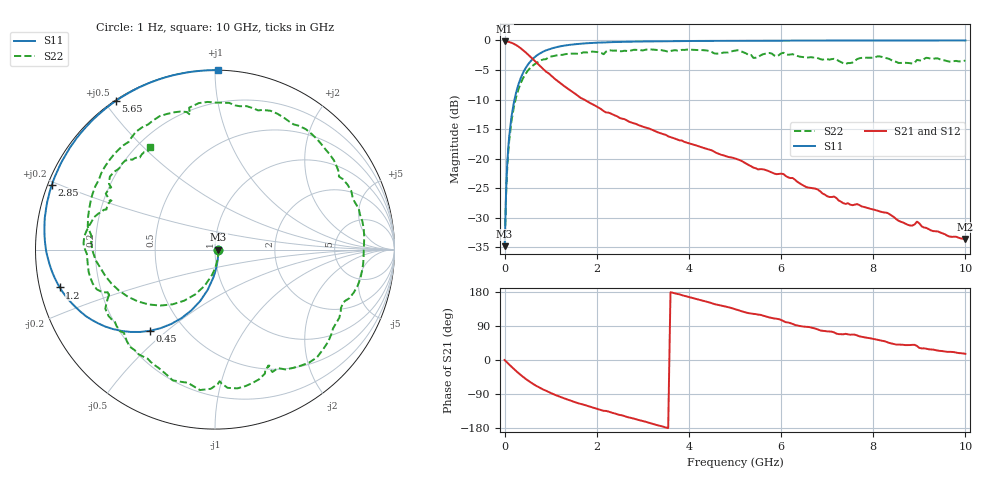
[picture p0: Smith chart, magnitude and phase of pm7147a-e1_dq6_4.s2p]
# GHz S DB R 50
! S-Parameters data
! Freq  dbS11  angS11  dbS21  angS21  dbS12  angS12  dbS22  angS22
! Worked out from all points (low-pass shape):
!   279 points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, 1 Hz to 10 GHz, reference 50 ohm
!   highest |S21| = -0.16 dB at 79.4 Hz (marker M1); lowest = -33.6 dB at 10 GHz (marker M2)
!   |S21| within 3 dB of the highest: start of sweep to 612.8 MHz
!   lowest |S11| = -34.8 dB at 79.4 Hz (marker M3), VSWR 1.04, Z = 51.9 - j3.07e-06 ohm
!   |S11| at or under -10 dB: start of sweep to 215.3 MHz
!   |S22| runs from -34.8 to -1.5 dB; largest |S21 - S12| = 1.1e-11
!   S11 on the Smith chart (normalised r, x): 1 Hz: 1.04, -0.00; 450 MHz: 0.32, -0.44; 1.2 GHz: 0.06, -0.12; 2.85 GHz: 0.01, +0.19; 5.65 GHz: 0.00, +0.54; 10 GHz: 0.00, +1.02
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1e-09  -34.81 -0.0  -0.16 -0.0  -0.16 -0.0  -34.81 -0.0
7.94e-08  -34.81 -0.0  -0.16 -0.0  -0.16 -0.0  -34.81 -0.0
0.03162278  -25.64 -72.5  -0.17 -3.8  -0.17 -3.8  -26.27 -72.2
0.06309573  -20.08 -85.6  -0.20 -7.6  -0.20 -7.6  -20.78 -87.2
0.15  -12.86 -100.2  -0.39 -17.8  -0.39 -17.8  -13.59 -105.9
0.3  -7.44 -116.0  -1.04 -34.4  -1.04 -34.4  -8.26 -127.8
0.45  -4.75 -128.6  -1.98 -49.1  -1.98 -49.1  -5.71 -146.2
0.8  -2.05 -150.3  -4.54 -75.6  -4.54 -75.6  -3.32 -179.5
1.2  -1.01 -166.3  -7.18 -97.0  -7.18 -97.0  -2.45 152.2
1.7  -0.52 179.9  -9.90 -117.4  -9.90 -117.4  -2.04 123.9
2.3  -0.29 167.6  -12.35 -138.0  -12.35 -138.0  -1.68 92.9
2.85  -0.19 158.4  -14.12 -156.2  -14.12 -156.2  -1.59 65.3
3.35  -0.14 151.0  -15.62 -173.0  -15.62 -173.0  -1.61 39.6
4.2  -0.08 139.8  -17.87 160.0  -17.87 160.0  -1.63 -2.6
5.05  -0.05 130.0  -20.10 132.2  -20.10 132.2  -1.65 -46.6
5.35  -0.04 126.8  -21.28 122.5  -21.28 122.5  -2.46 -64.9
5.65  -0.04 123.6  -21.88 115.6  -21.88 115.6  -2.25 -74.1
6.05  -0.03 119.7  -22.60 102.8  -22.60 102.8  -2.08 -96.1
6.7  -0.02 113.6  -25.02 84.3  -25.02 84.3  -2.89 -128.7
7.8  -0.01 104.3  -28.17 60.2  -28.17 60.2  -2.92 -169.9
8.35  -0.01 100.2  -29.38 45.0  -29.38 45.0  -3.14 164.9
10  -0.00 89.1  -33.59 16.3  -33.59 16.3  -3.40 122.1
